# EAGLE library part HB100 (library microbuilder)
HB100 Miniature Microwave Motion Sensor
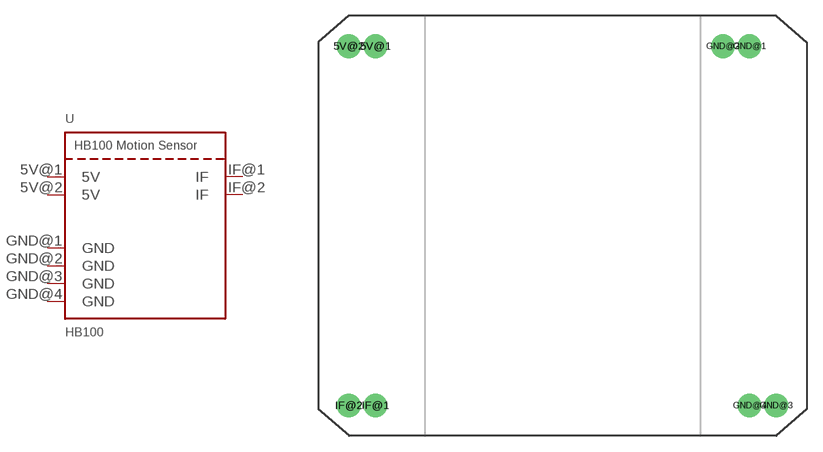
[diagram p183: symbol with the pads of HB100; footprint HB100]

Designator prefix U

## HB100  [HB100]
5V@1  5V
5V@2  5V
GND@1  GND
GND@2  GND
GND@3  GND
GND@4  GND
IF@1  IF
IF@2  IF

## Footprint HB100 (pad centres in mm)
drill 1.5: 5V@1 -17.81,15.83; 5V@2 -20.35,15.83; GND@1 17.81,15.83; GND@2 15.27,15.83; GND@3 20.35,-18.37; GND@4 17.81,-18.37; IF@1 -17.81,-18.37; IF@2 -20.35,-18.37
